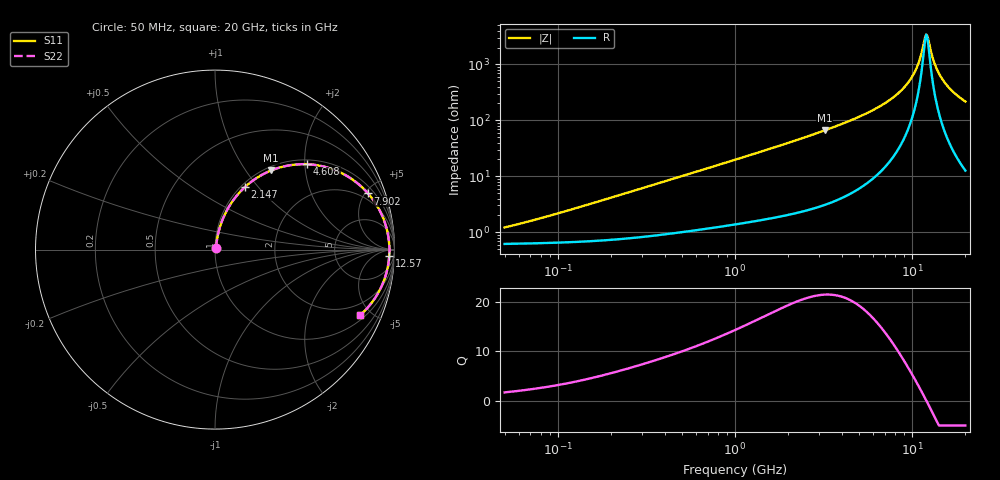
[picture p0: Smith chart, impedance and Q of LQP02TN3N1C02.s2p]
!Murata Part Number: LQP02TN3N1C02
!These Parameters are Measured in Series Mode Connection
!  o--[Z]--o
!Port1  Port2
!  o-------o
!Freq. Start=50[MHz] Stop=20[GHz], 401[Steps]
# Hz S RI R 50
!Freq.(Hz) S11(Real) S11(Imag) S21(Real) S21(Imag) S12(Real) S12(Imag) S22(Real) S22(Imag)
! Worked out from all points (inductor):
!   401 points, 50 MHz to 20 GHz, reference 50 ohm
!   read as one part in series: L = 3.28 nH near 93.8 MHz
!   highest Q = 21.5 at 3.217 GHz (marker M1), where L = 3.27 nH
!   self-resonance near 12.02 GHz
!   S11 on the Smith chart (normalised r, x): 50 MHz: 1.01, +0.02; 2.147 GHz: 1.04, +0.85; 4.608 GHz: 1.10, +2.06; 7.902 GHz: 1.46, +5.24; 12.57 GHz: 27, -34; 20 GHz: 1.25, -4.32
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5e7  0.00624 0.0103  0.9938 -0.0103  0.9938 -0.0103  0.00624 0.0103
1.364002e8  0.0075 0.0277  0.9925 -0.0277  0.9925 -0.0277  0.0075 0.0277
3.721004e8  0.0142 0.0732  0.9858 -0.0732  0.9858 -0.0732  0.0142 0.0732
1e9  0.0493 0.1843  0.9507 -0.1843  0.9507 -0.1843  0.0493 0.1843
2.146657e9  0.1658 0.3476  0.8342 -0.3476  0.8342 -0.3476  0.1658 0.3476
2.728004e9  0.243 0.4059  0.757 -0.4059  0.757 -0.4059  0.243 0.4059
3.216634e9  0.3128 0.441  0.6872 -0.441  0.6872 -0.441  0.3128 0.441
4.608136e9  0.5136 0.4756  0.4864 -0.4756  0.4864 -0.4756  0.5136 0.4756
5.856089e9  0.6711 0.4416  0.3289 -0.4416  0.3289 -0.4416  0.6711 0.4416
7.442007e9  0.8206 0.3461  0.1794 -0.3461  0.1794 -0.3461  0.8206 0.3461
7.901521e9  0.853 0.3126  0.147 -0.3126  0.147 -0.3126  0.853 0.3126
9.178299e9  0.9196 0.2142  0.0804 -0.2142  0.0804 -0.2142  0.9196 0.2142
1.019291e10  0.9512 0.1354  0.0488 -0.1354  0.0488 -0.1354  0.9512 0.1354
1.098561e10  0.9652 0.0757  0.0348 -0.0757  0.0348 -0.0757  0.9652 0.0757
1.183995e10  0.9714 0.0145  0.0286 -0.0145  0.0286 -0.0145  0.9714 0.0145
1.220001e10  0.9717 -0.0101  0.0283 0.0101  0.0283 0.0101  0.9717 -0.0101
1.257102e10  0.9708 -0.0348  0.0292 0.0348  0.0292 0.0348  0.9708 -0.0348
1.314879e10  0.967 -0.0716  0.033 0.0716  0.033 0.0716  0.967 -0.0716
1.354865e10  0.9629 -0.0959  0.0371 0.0959  0.0371 0.0959  0.9629 -0.0959
1.482269e10  0.9433 -0.1669  0.0567 0.1669  0.0567 0.1669  0.9433 -0.1669
1.696185e10  0.895 -0.2648  0.105 0.2648  0.105 0.2648  0.895 -0.2648
2e10  0.8105 -0.3638  0.1895 0.3638  0.1895 0.3638  0.8105 -0.3638
